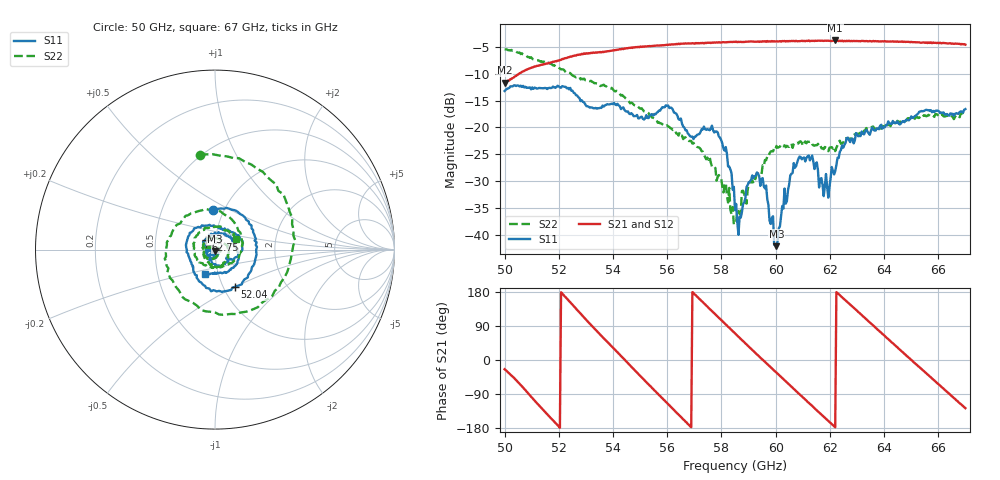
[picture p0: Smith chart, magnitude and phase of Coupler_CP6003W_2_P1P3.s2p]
!Agilent Technologies,E8361A,US42410132,A.06.03.05
!Agilent E8361A: A.06.03.05
!Date: Friday, July 11, 2008 16:49:03
!Correction: S11(Full 2 Port(1,2)) S21(Full 2 Port(1,2)) S12(Full 2 Port(1,2)) S22(Full 2 Port(1,2))
!S2P File: Measurements: S11, S21, S12, S22:
# Hz S  MA  R 50
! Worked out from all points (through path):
!   401 points, 50 GHz to 67 GHz, reference 50 ohm
!   highest |S21| = -3.80 dB at 62.2 GHz (marker M1); lowest = -11.7 dB at 50 GHz (marker M2)
!   lowest |S11| = -42.1 dB at 60.03 GHz (marker M3), VSWR 1.02, Z = 49.8 - j0.742 ohm
!   |S11| at or under -10 dB: start of sweep to end of sweep
!   |S22| runs from -38.1 to -5.5 dB; largest |S21 - S12| = 0.012
!   S11 on the Smith chart (normalised r, x): 50 GHz: 0.89, +0.41; 52.04 GHz: 1.14, -0.50; 62.75 GHz: 0.90, +0.10; 67 GHz: 0.86, -0.24
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5e10  0.2183 92.3  0.2611 -24.4  0.2645 -24.1  0.5336 99.2
5.08925e10  0.2336 17.7  0.3519 -90.0  0.3494 -90.1  0.4515 14.0
5.204e10  0.2355 -61.6  0.4239 -178.9  0.4209 -178.8  0.352 -89.3
5.28475e10  0.1786 -128.5  0.4845 118.8  0.483 118.7  0.2843 -161.6
5.357e10  0.1517 -171.2  0.4992 63.9  0.5083 63.6  0.2451 138.6
5.442e10  0.1458 114.4  0.5445 1.6  0.5389 1.2  0.192 60.9
5.5695e10  0.1433 39.5  0.5779 -92.4  0.5818 -91.9  0.1113 -46.6
5.70125e10  0.08176 -34.1  0.602 173.1  0.6103 174.0  0.06853 -154.9
5.7905e10  0.08209 -88.0  0.6213 111.3  0.6176 111.8  0.03592 155.6
5.85e10  0.01693 -141.3  0.6248 70.3  0.6292 70.7  0.01288 75.9
5.867e10  0.01479 -70.5  0.625 58.7  0.6299 58.6  0.0156 55.1
5.93075e10  0.03797 -100.8  0.628 14.7  0.632 15.4  0.03723 -55.8
6.003e10  0.00781 -107.4  0.6337 -33.3  0.6349 -33.2  0.06713 -131.7
6.0625e10  0.0376 -79.4  0.6362 -73.1  0.6385 -73.4  0.0644 168.2
6.13475e10  0.05462 -165.3  0.6384 -121.1  0.6427 -121.3  0.06964 112.8
6.18575e10  0.0367 169.0  0.6407 -155.1  0.6352 -155.3  0.06443 70.1
6.21975e10  0.03894 -175.3  0.6453 -177.6  0.6372 -177.5  0.06001 36.8
6.275e10  0.07288 132.5  0.6344 146.4  0.6353 146.2  0.07885 -16.2
6.4195e10  0.1096 38.7  0.6312 52.3  0.6324 52.4  0.1059 -128.1
6.53e10  0.1399 -17.8  0.6192 -18.5  0.618 -18.7  0.1227 157.5
6.6235e10  0.1324 -75.9  0.6098 -78.6  0.61 -78.5  0.1261 90.3
6.7e10  0.148 -112.1  0.59 -127.1  0.5849 -127.4  0.1298 28.0
